FUNCTION_BLOCK FB_CylinderDiag EXTENDS FB_Cylinder
(* FB_CylinderDiag	- number of control signals
							one direction is controllable
					- type of feedback signal
							feedback in base and work position
					- with diagnosis									*)
VAR_INPUT
	tTimeOut 	 	: TIME;
END_VAR
VAR_OUTPUT
	bError			: BOOL;
	sErrorMsg		: STRING;
END_VAR
VAR
	fbTriggerError	: R_TRIG;
	bErrorMove		: BOOL;
	fbTimerWatchDog	: TON;
END_VAR

// =========================================================
;
// =========================================================

METHOD M_StateMachine : BOOL
VAR_INPUT
	bBasePosReq		: BOOL;
	bWorkPosReq		: BOOL;
END_VAR
// =========================================================
	// Call the method M_StateMachine of base class FB_Cylinder via 'SUPER^.'

SUPER^.M_StateMachine(	bBasePosReq := bBasePosReq,
						bWorkPosReq	:= bWorkPosReq );

// =========================================================
	// Additional diagnosis

M_StateMachine := M_Diag();

// =========================================================
END_METHOD

METHOD PUBLIC M_Reset
VAR_INPUT
END_VAR
// =========================================================
	// Reset
	
SUPER^.M_Reset();		// Calling method M_Reset of base class FB_Cylinder via 'SUPER^.'

bError 		:= FALSE;
sErrorMsg 	:= '';

// =========================================================
END_METHOD

METHOD M_Diag : BOOL
VAR_INPUT
END_VAR
// =========================================================
	// Timer starts when cylinder is not in base and work position
	
IF NOT bAtBasePos AND NOT bAtWorkPos THEN
	fbTimerWatchDog(IN := TRUE, PT := tTimeOut);
ELSE
	fbTimerWatchDog(IN := FALSE, PT := tTimeOut);
END_IF

// =========================================================
	// Error if cylinder does not reach base or work position
	
fbTriggerError( CLK := fbTimerWatchDog.Q );

bError := fbTimerWatchDog.Q;

IF fbTriggerError.Q THEN
	bErrorMove := bMoveToWork;
END_IF

IF bError THEN
	
	IF bErrorMove = bMoveToWork THEN
		
		IF bMoveToWork THEN
			sErrorMsg := 'Work position not reached';
		ELSE
			sErrorMsg := 'Base position not reached';
		END_IF
		
	ELSE
		bError := FALSE;
		sErrorMsg := '';
	END_IF
	
ELSE
	sErrorMsg := '';
END_IF

// =========================================================
	// Return
	
M_Diag := bError;

// =========================================================
END_METHOD

END_FUNCTION_BLOCK
